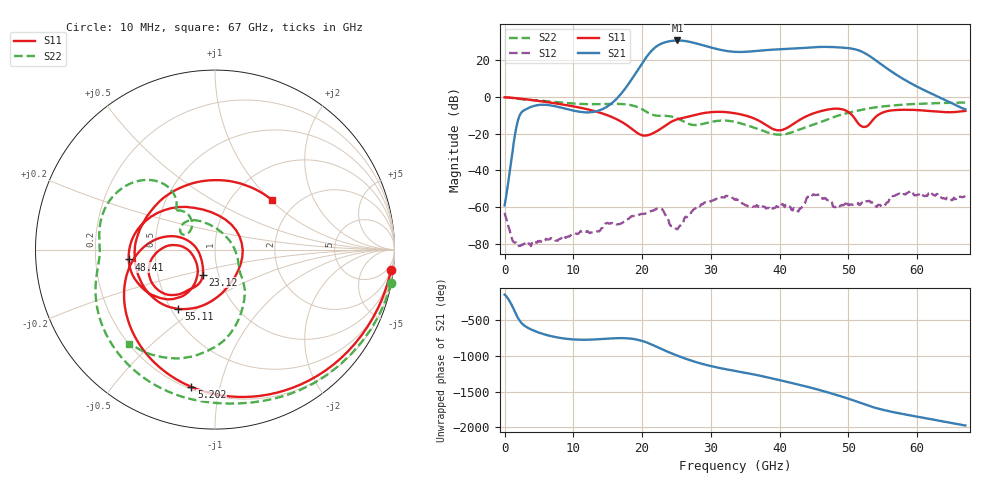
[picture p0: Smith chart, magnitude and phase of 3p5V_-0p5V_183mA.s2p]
! MARKI MICROWAVE INC.
! Date:  10/23/18
! Model Number:  AMM-6702CH
! Description:  2-port Small Signal S-parameter data for AMM-6702CH
! Frequency Range:  10 MHz to 67 GHz
! Port Configuration:  PORT 1: Input
!  PORT 2: Output
! Bias Condition: Vd = +3.5V, Vg = -0.5V
! AMM-6702CH s2p files are only valid for small signal conditions (below -5 dBm input power)
!S2P File: Measurements: Mag<S11> Ang<S11>, Mag<S21> Ang<S21>, Mag<S12> Ang<S12>, Mag<S22> Ang<S22>!row 1
# Hz S  dB  R 50
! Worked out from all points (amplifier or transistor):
!   401 points, 10 MHz to 67 GHz, reference 50 ohm
!   highest |S21| = 30.9 dB at 25.13 GHz (marker M1)
!   |S21| within 3 dB of that: 22.18 GHz to 29.2 GHz (7.016 GHz wide, 27.3 % of centre)
!   unconditionally stable (mu >= 1): start of sweep to end of sweep
!   at 11.06 GHz: K = 2396.32, MAG = -4.3 dB, |S12| = -73.0 dB
!   at 33.51 GHz: K = 15.24, MAG = 25.5 dB, |S12| = -56.0 dB
!   at 67 GHz: K = 227.61, MAG = -2.7 dB, |S12| = -54.3 dB
!   S11 on the Smith chart (normalised r, x): 10 MHz: 2, -17; 5.202 GHz: 0.21, -0.82; 23.12 GHz: 0.84, -0.24; 48.41 GHz: 0.35, -0.05; 55.11 GHz: 0.55, -0.42; 67 GHz: 1.50, +1.02
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1e7  -0.11 -6.7  -59.01 -146.6  -63.11 -126.6  -0.02 -10.8
5.201725e9  -2.20 -99.8  -4.20 35.9  -78.36 108.6  -1.95 -128.8
1.123082e10  -5.95 -165.4  -8.15 -57.0  -73.33 172.7  -3.74 -174.2
1.993952e10  -20.74 -171.2  18.07 -71.7  -63.71 135.9  -6.46 128.6
2.14468e10  -19.93 -135.8  25.54 -126.2  -61.92 122.7  -9.52 129.7
2.245165e10  -17.88 -121.5  28.52 -170.7  -60.84 92.1  -10.21 135.6
2.312155e10  -16.23 -115.9  29.63 160.3  -62.36 66.6  -10.20 136.4
2.513125e10  -12.10 -120.4  30.89 81.2  -72.02 100.5  -11.60 128.4
2.630358e10  -11.01 -124.7  30.55 39.3  -65.24 135.4  -13.84 129.4
2.74759e10  -9.89 -128.9  29.65 1.8  -61.26 127.3  -15.21 141.2
2.982055e10  -8.28 -143.0  27.24 -60.0  -56.88 108.0  -13.66 154.6
3.3505e10  -8.81 -170.2  24.67 -131.2  -55.99 33.9  -13.51 129.2
3.718945e10  -13.31 173.5  25.35 160.1  -59.56 10.7  -17.81 93.9
4.037148e10  -17.88 -144.1  26.17 91.1  -58.29 -19.9  -20.39 31.6
4.472582e10  -9.11 -129.0  27.15 -10.5  -53.62 12.6  -15.21 -38.4
4.673552e10  -6.97 -148.7  27.39 -64.1  -55.41 166.9  -12.50 -48.6
4.841028e10  -6.30 -173.5  27.16 -111.2  -58.71 147.8  -10.21 -57.8
5.02525e10  -8.85 142.8  26.57 -167.3  -58.48 -169.3  -8.31 -68.1
5.209472e10  -16.19 28.3  24.53 130.1  -57.83 -37.9  -6.79 -77.4
5.510928e10  -8.22 -121.6  16.94 43.3  -59.56 59.0  -5.05 -93.1
5.594665e10  -7.42 -135.6  14.73 25.1  -55.84 22.1  -4.74 -96.7
6.7e10  -7.52 41.5  -6.64 -172.4  -54.34 -14.6  -2.96 -132.5
